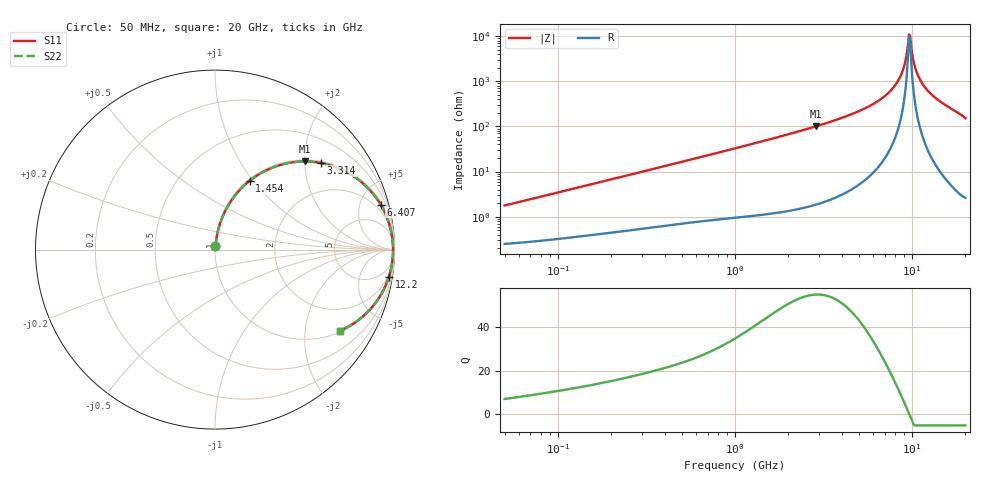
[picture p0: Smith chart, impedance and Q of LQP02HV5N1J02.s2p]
!Murata Part Number: LQP02HV5N1J02
!These Parameters are Measured in Series Mode Connection
!  o--[Z]--o
!Port1  Port2
!  o-------o
!Freq. Start=50[MHz] Stop=20[GHz], 401[Steps]
# Hz S RI R 50
!Freq.(Hz) S11(Real) S11(Imag) S21(Real) S21(Imag) S12(Real) S12(Imag) S22(Real) S22(Imag)
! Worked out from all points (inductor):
!   401 points, 50 MHz to 20 GHz, reference 50 ohm
!   read as one part in series: L = 5.53 nH near 51.52 MHz
!   highest Q = 54.5 at 2.853 GHz (marker M1), where L = 5.6 nH
!   self-resonance near 9.6 GHz
!   S11 on the Smith chart (normalised r, x): 50 MHz: 1.00, +0.04; 1.454 GHz: 1.02, +0.96; 3.314 GHz: 1.04, +2.41; 6.407 GHz: 1.24, +7.28; 12.2 GHz: 2, -13; 20 GHz: 1.05, -3.06
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5e7  0.00278 0.0174  0.9972 -0.0174  0.9972 -0.0174  0.00278 0.0174
1.364002e8  0.00578 0.0458  0.9942 -0.0458  0.9942 -0.0458  0.00578 0.0458
3.721004e8  0.0206 0.1196  0.9794 -0.1196  0.9794 -0.1196  0.0206 0.1196
1e9  0.1034 0.2904  0.8966 -0.2904  0.8966 -0.2904  0.1034 0.2904
1.454215e9  0.1925 0.3829  0.8075 -0.3829  0.8075 -0.3829  0.1925 0.3829
2.728004e9  0.4757 0.4903  0.5243 -0.4903  0.5243 -0.4903  0.4757 0.4903
2.853386e9  0.5017 0.4909  0.4983 -0.4909  0.4983 -0.4909  0.5017 0.4909
3.314454e9  0.5904 0.4826  0.4096 -0.4826  0.4096 -0.4826  0.5904 0.4826
4.81993e9  0.8028 0.3868  0.1972 -0.3868  0.1972 -0.3868  0.8028 0.3868
6.406762e9  0.9227 0.2508  0.0773 -0.2508  0.0773 -0.2508  0.9227 0.2508
7.442007e9  0.9634 0.1643  0.0366 -0.1643  0.0366 -0.1643  0.9634 0.1643
8.644534e9  0.9867 0.0714  0.0133 -0.0714  0.0133 -0.0714  0.9867 0.0714
9.041845e9  0.9901 0.0428  0.0099 -0.0428  0.0099 -0.0428  0.9901 0.0428
9.457416e9  0.9918 0.0139  0.00815 -0.0139  0.00815 -0.0139  0.9918 0.0139
9.600142e9  0.9921 0.00428  0.00795 -0.00428  0.00795 -0.00428  0.9921 0.00428
9.892087e9  0.9919 -0.0151  0.00811 0.0151  0.00811 0.0151  0.9919 -0.0151
1.034674e10  0.9902 -0.0442  0.00978 0.0442  0.00978 0.0442  0.9902 -0.0442
1.066139e10  0.9881 -0.0636  0.0119 0.0636  0.0119 0.0636  0.9881 -0.0636
1.131968e10  0.9816 -0.1024  0.0184 0.1024  0.0184 0.1024  0.9816 -0.1024
1.220001e10  0.969 -0.1506  0.031 0.1506  0.031 0.1506  0.969 -0.1506
1.460232e10  0.9168 -0.2633  0.0832 0.2633  0.0832 0.2633  0.9168 -0.2633
2e10  0.6978 -0.4507  0.3022 0.4507  0.3022 0.4507  0.6978 -0.4507
